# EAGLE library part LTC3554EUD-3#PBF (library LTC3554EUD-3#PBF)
Battery Management Micropower USB Power Manager with Li-Ion Charger and Two Step Down Regulators Source: Datasheet
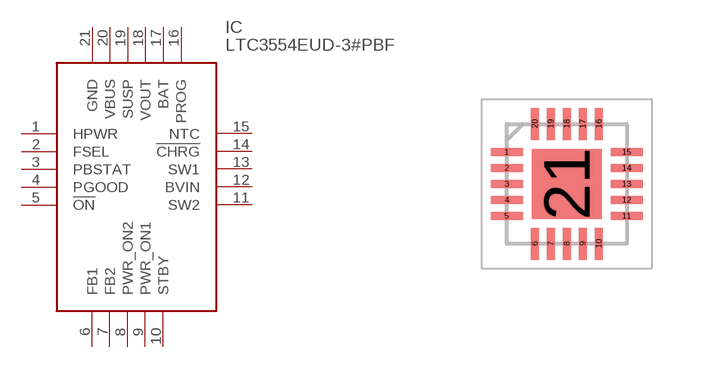
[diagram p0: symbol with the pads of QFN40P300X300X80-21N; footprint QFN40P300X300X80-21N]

Designator prefix IC

## LTC3554EUD-3#PBF (Description: Battery Management Micropower USB Power Manager with Li-Ion Charger and Two Step Down Regulators; Height: 0.8mm; Manufacturer_Name: Analog Devices; Manufacturer_Part_Number: LTC3554EUD-3#PBF; Mouser_Part_Number: 584-LTC3554EUD-3#PBF; Mouser_Price-Stock: https://www.mouser.com/Search/Refine.aspx?Keyword=584-LTC3554EUD-3%23PBF)  [QFN40P300X300X80-21N]
1  HPWR
2  FSEL
3  PBSTAT
4  PGOOD
5  !ON
6  FB1
7  FB2
8  PWR_ON2
9  PWR_ON1
10  STBY
11  SW2
12  BVIN
13  SW1
14  !CHRG
15  NTC
16  PROG
17  BAT
18  VOUT
19  SUSP
20  VBUS
21  GND

## Footprint QFN40P300X300X80-21N (pad centres in mm)
UD Package 20-Lead Plastic QFN (3mm &times; 3mm)
smd 0.8 x 0.2: 1 -1.5,0.8; 2 -1.5,0.4; 3 -1.5,0; 4 -1.5,-0.4; 5 -1.5,-0.8; 11 1.5,-0.8; 12 1.5,-0.4; 13 1.5,0; 14 1.5,0.4; 15 1.5,0.8
smd 0.2 x 0.8: 6 -0.8,-1.5; 7 -0.4,-1.5; 8 0,-1.5; 9 0.4,-1.5; 10 0.8,-1.5; 16 0.8,1.5; 17 0.4,1.5; 18 0,1.5; 19 -0.4,1.5; 20 -0.8,1.5
smd 1.75 x 1.75: 21 0,0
